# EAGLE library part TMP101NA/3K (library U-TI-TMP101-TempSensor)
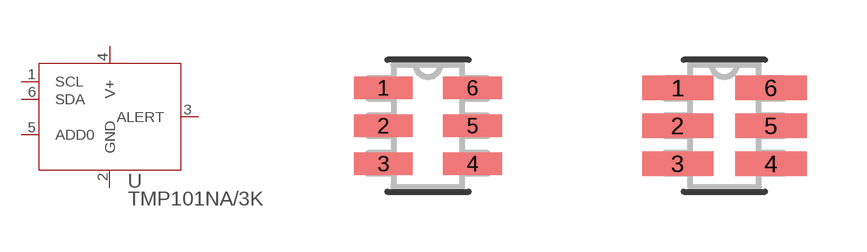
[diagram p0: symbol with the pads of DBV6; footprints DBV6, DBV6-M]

Designator prefix U

## TMP101NA/3K (MANUFACTURER_PART_NUMBER: TMP101NA3K; VENDOR: Texas Instruments)  [DBV6]
1  SCL  in
2  GND  pwr
3  ALERT  out
4  V+  pwr
5  ADD0  in
6  SDA  oc

## TMP101NA/3KDBV6-M (MANUFACTURER_PART_NUMBER: TMP101NA3K; VENDOR: Texas Instruments)  [DBV6-M]
Pads as for DBV6

## TMP101NA/3KDBV6-L (MANUFACTURER_PART_NUMBER: TMP101NA3K; VENDOR: Texas Instruments)  [DBV6-L]
Pads as for DBV6

## TMP101NA/3KSLOTTED  [DBV6-SLOT]
1  SDA  oc
2  ADD0  in
3  V+  pwr
4  ALERT  out
5  GND  pwr
6  SCL  in

## Footprint DBV6 (pad centres in mm)
smd 1.473 x 0.559: 1 -1.118,0.95; 2 -1.118,0; 3 -1.118,-0.95; 4 1.118,-0.95; 5 1.118,0; 6 1.118,0.95

## Footprint DBV6-M (pad centres in mm)
smd 1.778 x 0.61: 1 -1.168,0.95; 2 -1.168,0; 3 -1.168,-0.95; 4 1.168,-0.95; 5 1.168,0; 6 1.168,0.95

## Footprint DBV6-L (pad centres in mm)
smd 1.168 x 0.508: 1 -1.067,0.95; 2 -1.067,0; 3 -1.067,-0.95; 4 1.067,-0.95; 5 1.067,0; 6 1.067,0.95

## Footprint DBV6-SLOT (pad centres in mm)
**README I AM IMPORTANT** This variant of the chip is specifically designed to be soldered upside down with the package fitting inside the board so that it will be able to get a more accurate reading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
smd 1.1 x 0.6: 1 1.75,0.95; 2 1.75,0; 3 1.75,-0.95; 4 -1.75,-0.95; 5 -1.75,0; 6 -1.75,0.95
